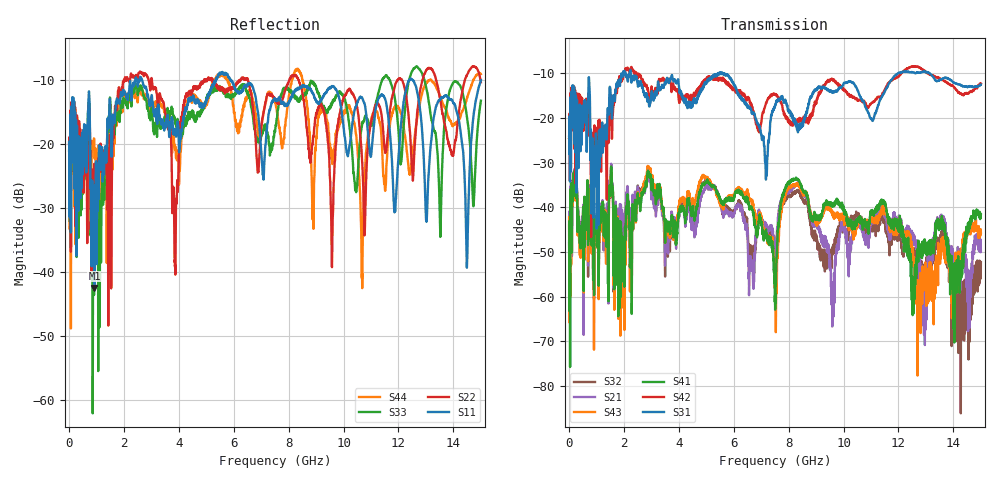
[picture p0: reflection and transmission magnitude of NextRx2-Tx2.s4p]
! FILE: N:\QM 2007\Prüfprotokolle\Highspeed\Konfektionierte Ltg\L45593-D106\D30\8216\0002\Next  Platine 2\NextRx2-Tx2.s4p
# MHz S DB R 50.00
! FREQ  S11  S12  S13  S14
!  S21  S22  S23  S24
!  S31  S32  S33  S34
!  S41  S42  S43  S44
!  DB  ANG  DB  ANG  DB  ANG  DB  ANG
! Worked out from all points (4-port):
!   2999 points, 10 MHz to 15 GHz, reference 50 ohm
!   strongest paths, dB at 10 MHz, 3.755 GHz, 7.505 GHz, 11.26 GHz, 15 GHz:
!     S31: -24.2, -10.4, -17.3, -17.1, -12.5
!     S42: -24.7, -13.2, -14.7, -15.4, -12.3
!     S41: -47.7, -42.3, -59.7, -40.5, -41.6
!     S43: -42.2, -42.9, -58.1, -43.0, -45.7
!     S21: -48.1, -41.3, -50.0, -41.7, -49.8
!     S32: -44.0, -43.5, -50.0, -44.4, -52.3
!   lowest |S11| = -42.4 dB at 930 MHz (marker M1), VSWR 1.02, Z = 50.2 + j0.72 ohm
!   |S11| at or under -10 dB: 2.667 GHz to 5.334 GHz (2.667 GHz wide, 66.7 % of centre); 5.892 GHz to 12.4 GHz (6.507 GHz wide, 71.1 % of centre); 12.52 GHz to end of sweep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
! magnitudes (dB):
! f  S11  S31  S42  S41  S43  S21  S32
! 10 MHz  -19.7  -24.2  -24.7  -47.7  -42.2  -48.1  -44.0
! 930 MHz  -42.4  -35.0  -21.7  -45.2  -45.9  -45.8  -46.0
! 2.415 GHz  -10.1  -11.2  -10.2  -38.4  -38.8  -37.1  -38.1
! 3.83 GHz  -18.4  -11.4  -13.2  -45.1  -44.7  -43.0  -43.3
! 10.66 GHz  -12.7  -15.8  -16.1  -43.7  -43.0  -44.6  -43.1
! 14.49 GHz  -38.7  -13.1  -14.5  -46.4  -46.5  -55.1  -67.4
! 15 GHz  -10.0  -12.5  -12.3  -41.6  -45.7  -49.8  -52.3
